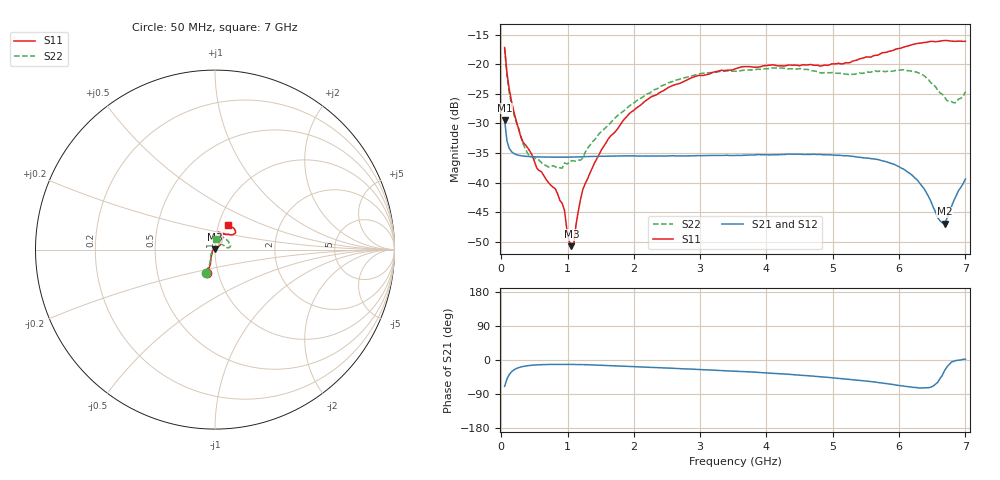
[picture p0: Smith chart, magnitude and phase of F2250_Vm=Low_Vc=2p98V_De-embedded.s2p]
! Integrated Device Technology
! Corporate Headquarters
! 6024 Silver Creek Valley Road
! San Jose, CA 95138  USA
! Phone:  1-408-284-8200
! Toll Free:  1-800-223-1366
! Webpage:  http://www.idt.com/
! Timing and RF Division
! 515 Groton Road, Suite 102
! Westford, MA 01886-6024
! Device:  F2250
! Description: Voltage Variable RF Attenuator
! Frequency:  50.0 -  6000.00 MHz
! Package:  3x3 mm Thin QFN Plastic Package: 16 pin
! Ports:  2 RF, 3 DC
!  Pin  1  = GND
!  Pin  2  = NC
!  Pin  3  = RF1  = Port 1
!  Pin  4  = NC
!  Pin  5  = GND
!  Pin  6  = GND
!  Pin  7  = GND
!  Pin  8  = GND
!  Pin  9  = NC
!  Pin 10  = RF2  = Port 2
!  Pin 11  = NC
!  Pin 12  = GND
!  Pin 13  = GND
!  Pin 14  = VCNTRL
!  Pin 15  = VDD
!  Pin 16  = VMODE
! Vcntrl:  2.980 Volts
! Vmode:  +0.000 Volts
! Vdd:  +3.30  Volts
! Current:  1.176 mA
! Data:  The device was measured on a the F2250 evaluation board which has
!  individual transmission lines to the RF pins.  Data was collected
!  using a calibrated network analyzer.  The evaluation board was
!  de-embedded using a TRL calibration technique.
!  The reference plane is the edge of the package pin.
! Misc:  SN 10
!  Action Tracker AT0258
! Date Measured:  2014-11-26
! Date:  2015-10-15  MJV
! Note:
!  Integrated Device Technology supplies this data as a sample of measured
!  data at the package pin for this product.  Your particular data for this
!  product may vary.
!  Data was taken at 25 degrees C.
!  Integrated Device Technology reserves the right to change this data at anytime.
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# GHz S dB R 50
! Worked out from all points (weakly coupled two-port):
!   201 points, 50 MHz to 7 GHz, reference 50 ohm
!   highest |S21| = -29.42 dB at 50 MHz (marker M1); lowest = -46.9 dB at 6.687 GHz (marker M2)
!   lowest |S11| = -50.7 dB at 1.058 GHz (marker M3), VSWR 1.01, Z = 49.8 + j0.24 ohm
!   |S11| at or under -10 dB: start of sweep to end of sweep
!   |S22| runs from -37.5 to -17.3 dB; largest |S21 - S12| = 7.7e-05
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0.05  -17.18 -108.6  -29.42 -69.8  -29.41 -69.8  -17.28 -111.0
0.08475  -21.45 -107.5  -32.92 -50.4  -32.92 -50.3  -21.74 -110.2
0.15425  -26.23 -116.6  -34.76 -31.2  -34.76 -31.2  -26.82 -122.5
0.29325  -32.22 -127.9  -35.43 -18.5  -35.43 -18.5  -32.09 -137.4
0.3975  -34.10 -142.0  -35.56 -15.0  -35.56 -15.0  -35.05 -160.4
0.5365  -37.55 -155.6  -35.63 -12.8  -35.64 -12.8  -36.05 178.1
0.91875  -43.48 158.0  -35.69 -11.5  -35.69 -11.5  -37.54 133.7
1.023  -49.86 143.4  -35.67 -11.6  -35.67 -11.6  -36.65 116.0
1.05775  -50.70 124.3  -35.67 -11.7  -35.67 -11.6  -36.27 110.7
1.0925  -50.40 89.4  -35.66 -11.7  -35.65 -11.7  -36.29 106.5
1.162  -44.75 57.1  -35.64 -11.9  -35.64 -11.9  -36.19 95.4
1.2315  -41.07 44.4  -35.61 -12.1  -35.61 -12.1  -35.79 85.8
1.6485  -32.11 42.0  -35.52 -14.7  -35.51 -14.7  -29.87 64.5
1.9265  -28.39 41.3  -35.47 -16.9  -35.47 -16.9  -27.10 56.7
2.37825  -24.87 47.3  -35.48 -20.3  -35.48 -20.3  -23.99 56.8
3.525  -20.79 72.4  -35.40 -29.5  -35.40 -29.6  -21.19 74.7
4.7065  -20.17 72.3  -35.19 -42.6  -35.19 -42.7  -21.14 72.2
5.85325  -17.81 40.5  -36.63 -63.4  -36.63 -63.5  -21.14 23.1
6.27025  -16.50 40.0  -39.49 -72.8  -39.51 -72.9  -21.37 9.7
6.68725  -15.99 48.7  -46.90 -27.5  -46.87 -27.2  -25.63 28.7
6.861  -16.14 55.1  -42.20 -1.4  -42.16 -1.5  -26.44 57.9
7  -16.13 63.2  -39.38 1.9  -39.33 1.7  -24.64 83.0
